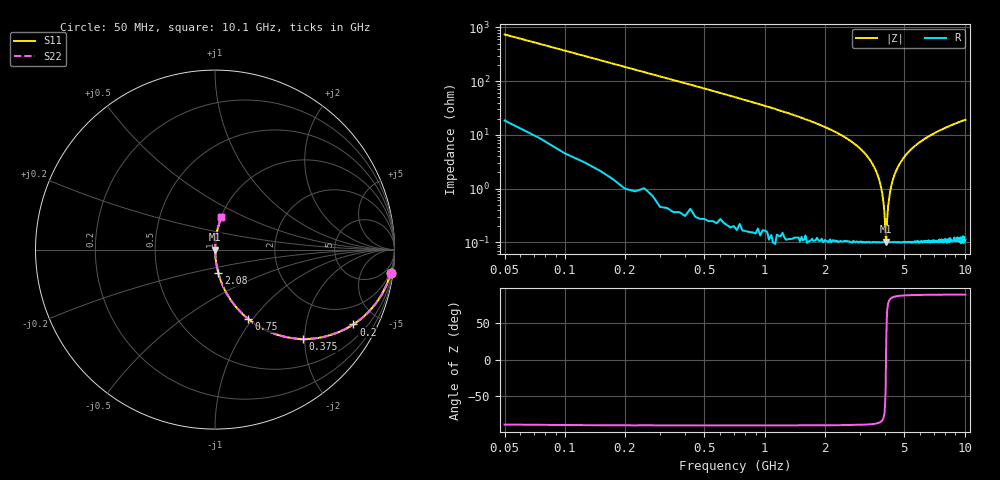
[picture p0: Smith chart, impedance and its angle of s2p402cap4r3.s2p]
! AVX Thin Film Operation		Date: April 2003
! Description: Accu-P® Series, Thin Film, SMD, RF Capacitor
! Part Number: 04025J4R3ABS
! 50 MHz  -  10.05 GHz
! Serial Measurements
# hz S db R 50
!	S11		S21		S12		S22
!	dB	Phase	dB	Phase	dB	Phase	dB	Phase
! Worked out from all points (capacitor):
!   400 points, 50 MHz to 10.1 GHz, reference 50 ohm
!   read as one part in series: C = 4.3 pF near 100 MHz
!   lowest |Z| = 102 mohm at 4.05 GHz (marker M1)
!   series resonance near 4.046 GHz, so ESL is about 360 pH
!   S11 on the Smith chart (normalised r, x): 50 MHz: 1, -15; 200 MHz: 1.02, -3.69; 375 MHz: 1.01, -1.96; 750 MHz: 1.00, -0.95; 2.08 GHz: 1.00, -0.26; 10.1 GHz: 1.00, +0.38
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5e7  -0.11 -7.7  -17.50 80.9  -17.50 80.9  -0.11 -7.7
1e8  -0.33 -15.1  -11.70 74.2  -11.70 74.2  -0.33 -15.1
2e8  -1.14 -28.4  -6.47 61.3  -6.47 61.3  -1.14 -28.4
3.75e8  -3.12 -45.5  -2.94 44.3  -2.94 44.3  -3.12 -45.5
7.5e8  -7.34 -64.3  -0.90 25.4  -0.90 25.4  -7.34 -64.3
1.73e9  -15.30 -79.7  -0.14 9.9  -0.14 9.9  -15.30 -79.7
2.08e9  -17.70 -82.1  -0.08 7.5  -0.08 7.5  -17.70 -82.1
2.88e9  -23.90 -85.4  -0.03 3.6  -0.03 3.6  -23.90 -85.4
3.4e9  -29.90 -86.4  -0.01 1.8  -0.01 1.8  -29.90 -86.4
3.68e9  -35.10 -85.7  -0.01 1.0  -0.01 1.0  -35.10 -85.7
3.88e9  -42.00 -82.3  -0.01 0.5  -0.01 0.5  -42.00 -82.3
3.98e9  -49.50 -72.5  -0.01 0.2  -0.01 0.2  -49.50 -72.5
4.05e9  -59.80 12.4  -0.01 -0.0  -0.01 -0.0  -59.80 12.4
4.1e9  -51.50 67.8  -0.01 -0.1  -0.01 -0.1  -51.50 67.8
4.15e9  -46.40 77.7  -0.01 -0.3  -0.01 -0.3  -46.40 77.7
4.3e9  -39.00 84.2  -0.01 -0.6  -0.01 -0.6  -39.00 84.2
4.6e9  -32.50 86.2  -0.01 -1.4  -0.01 -1.4  -32.50 86.2
5.08e9  -27.60 86.2  -0.02 -2.4  -0.02 -2.4  -27.60 86.2
5.85e9  -23.20 85.2  -0.03 -4.0  -0.03 -4.0  -23.20 85.2
6.75e9  -20.20 83.8  -0.05 -5.6  -0.05 -5.6  -20.20 83.8
8.43e9  -16.80 81.2  -0.10 -8.3  -0.10 -8.3  -16.80 81.2
1.01e10  -14.60 78.9  -0.16 -10.8  -0.16 -10.8  -14.60 78.9
